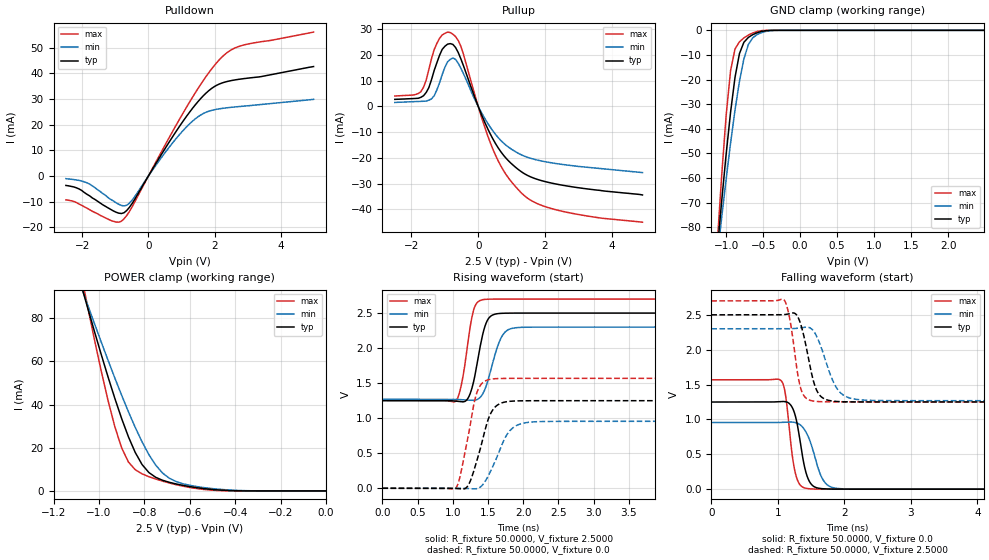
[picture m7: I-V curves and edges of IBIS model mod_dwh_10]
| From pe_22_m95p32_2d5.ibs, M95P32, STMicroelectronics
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|   Model mod_dwh_10
[Model]   mod_dwh_10
Model_type I/O
Polarity   Non-Inverting
Enable   Active-High
Vinl   =   0.750V
Vinh   =   1.750V
Vmeas  =   1.250V
Cref   =   30.0pF
C_comp   1.219pF   1.164pF   1.337pF
[Model Spec]
Vinl   0.750V  0.690V  0.810V  | <- for Vcc = 2.5V, 2.3V, 2.7V
Vinh   1.750V  1.610V  1.890V  | <- for Vcc = 2.5V, 2.3V, 2.7V
Vmeas  1.250V  1.150V  1.350V  | <- for Vcc = 2.5V, 2.3V, 2.7V
[Temperature Range]  25.0000   0.1050k   -40.0000
[Voltage Range]   2.5000V   2.3000V   2.7000V
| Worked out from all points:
|   slope of the pulldown table from 0 to 0.375 V, typ, clamps not added: 46.8 ohm
|   slope of the pullup table from 0 to 0.375 V, typ, clamps not added: 33.9 ohm
|   GND clamp passes 1 mA (typ) near -0.58 V on its own axis
|   POWER clamp passes 1 mA (typ) near -0.53 V on its own axis
|   rising waveform, R_fixture 50.0000, V_fixture 2.5000: 20-80 % time 148ps typ, 183ps min, 131ps max; typ from 1.25 V to 2.5 V
|   rising waveform, R_fixture 50.0000, V_fixture 0.0: 20-80 % time 210ps typ, 257ps min, 178ps max; typ from 0 V to 1.25 V
|   falling waveform, R_fixture 50.0000, V_fixture 0.0: 20-80 % time 144ps typ, 197ps min, 116ps max; typ from 1.25 V to 0 V
|   falling waveform, R_fixture 50.0000, V_fixture 2.5000: 20-80 % time 173ps typ, 240ps min, 135ps max; typ from 2.5 V to 1.25 V
[Pulldown]
|Voltage   I(typ)   I(min)   I(max)
-2.5V     -3.72mA    -1.07mA    -9.34mA
-1.86V    -7.2mA     -2.7mA     -12.6mA
-1.14V    -13.1mA    -9.2mA     -17.4mA
-820mV    -14.69mA   -11.52mA   -17.69mA
-660mV    -13.52mA   -11.47mA   -15.5mA
-500mV    -10.87mA   -9.532mA   -12.19mA
540mV     11.44mA    9.728mA    12.92mA
1.26V     25.15mA    20.5mA     29.15mA
1.74V     32.3mA     24.84mA    38.73mA
2.22V     36.25mA    26.34mA    46.35mA
2.86V     37.94mA    27.21mA    51.03mA
5V        42.7mA     29.9mA     56.16mA
[Pullup]
|Voltage   I(typ)   I(min)   I(max)
-2.5V     2.762mA    1.562mA    4.052mA
-1.72V    3.553mA    1.982mA    5.743mA
-1.48V    7.344mA    2.457mA    14.39mA
-1.24V    16.99mA    6.442mA    24.51mA
-1.08V    22.2mA     12.4mA     27.82mA
-840mV    24.44mA    18.28mA    28.74mA
-520mV    18.48mA    14.85mA    23.37mA
120mV     -3.865mA   -2.929mA   -5.077mA
520mV     -14.48mA   -10.9mA    -19.03mA
1.32V     -25.62mA   -18.96mA   -33.95mA
2.44V     -30.41mA   -22.38mA   -40.5mA
4.92V     -34.4mA    -25.7mA    -44.98mA
[GND_clamp]
|Voltage   I(typ)   I(min)   I(max)
-2.5V     -618.8mA   -507.1mA   -839.7mA
-1.12V    -89.51mA   -92.19mA   -86.51mA
-1.06V    -69.34mA   -76.02mA   -58.94mA
-1V       -50.38mA   -60.48mA   -34.64mA
-940mV    -33.28mA   -45.81mA   -16.38mA
-880mV    -19.11mA   -32.38mA   -7.564mA
-820mV    -9.453mA   -20.71mA   -4.67mA
-760mV    -4.854mA   -11.6mA    -3.093mA
-700mV    -2.891mA   -5.814mA   -1.933mA
-580mV    -964.2uA   -1.685mA   -447.5uA
-340mV    -4.19uA    -39.9uA    -134.6nA
2.48V     343.3pA    931.5nA    131.5pA
[POWER_clamp]
|Voltage   I(typ)   I(min)   I(max)
-2.49V    667.2mA    541mA      921mA
-1.08V    96.07mA    95.11mA    101.2mA
-1.05V    84.91mA    86.28mA    85.45mA
-990mV    63.23mA    68.98mA    55.57mA
-930mV    42.88mA    52.31mA    29.76mA
-900mV    33.53mA    44.31mA    19.96mA
-840mV    17.8mA     29.4mA     9.816mA
-810mV    12.22mA    22.72mA    7.905mA
-750mV    6.305mA    11.96mA    5.516mA
-660mV    3.226mA    4.34mA     2.89mA
-420mV    154.8uA    392.4uA    29.01uA
0V        492.2pA    14.11nA    240.5pA
[Ramp]
| variable   typ   min   max
dV/dt_r   0.7498/0.2355n   0.5900/0.3071n   0.9410/0.1910n
dV/dt_f   0.7496/0.2142n   0.6311/0.3208n   0.8690/0.1617n
R_load = 50.0000
[Rising Waveform]
R_fixture= 50.0000
V_fixture= 2.5000
V_fixture_min= 2.3000
V_fixture_max= 2.7000
|time   V(typ)   V(min)   V(max)
0s        1.251V     1.269V     1.252V
1.04ns    1.244V     1.268V     1.24V
1.136ns   1.233V     1.263V     1.547V
1.248ns   1.353V     1.256V     2.308V
1.312ns   1.597V     1.257V     2.59V
1.424ns   2.189V     1.345V     2.691V
1.52ns    2.438V     1.611V     2.699V
1.68ns    2.496V     2.132V     2.7V
1.872ns   2.5V       2.288V     2.7V
8ns       2.5V       2.3V       2.7V
[Rising Waveform]
R_fixture= 50.0000
V_fixture= 0.0
V_fixture_min= 0.0
V_fixture_max= 0.0
|time   V(typ)   V(min)   V(max)
0s        5.246nV    623.3nV    889pV
1.04ns    -2.183mV   587.5uV    -1.489mV
1.104ns   -7.264mV   -5.605nV   170.9mV
1.2ns     16.06mV    -2.904mV   644.9mV
1.344ns   399.9mV    -4.835mV   1.369V
1.424ns   692.4mV    48.27mV    1.506V
1.536ns   1.062V     240.9mV    1.556V
1.792ns   1.239V     797.6mV    1.568V
2.08ns    1.249V     941.7mV    1.568V
8ns       1.25V      955.1mV    1.568V
[Falling Waveform]
R_fixture= 50.0000
V_fixture= 0.0
V_fixture_min= 0.0
V_fixture_max= 0.0
|time   V(typ)   V(min)   V(max)
0s        1.25V      955.1mV    1.568V
1.056ns   1.258V     957.9mV    1.549V
1.12ns    1.253V     961.1mV    1.325V
1.216ns   1.173V     962.2mV    490.1mV
1.264ns   1.048V     955.2mV    228.3mV
1.424ns   235.5mV    817.6mV    12.35mV
1.52ns    53.72mV    586.1mV    2.853mV
1.664ns   7.123mV    161.3mV    372.6uV
1.888ns   595.9uV    11.41mV    22.35uV
8ns       1.028uV    1.623uV    1.112uV
[Falling Waveform]
R_fixture= 50.0000
V_fixture= 2.5000
V_fixture_min= 2.3000
V_fixture_max= 2.7000
|time   V(typ)   V(min)   V(max)
0s        2.5V       2.3V       2.7V
1.088ns   2.503V     2.299V     2.72V
1.184ns   2.519V     2.301V     2.418V
1.28ns    2.501V     2.306V     1.77V
1.344ns   2.365V     2.313V     1.447V
1.52ns    1.607V     2.286V     1.265V
1.648ns   1.329V     2.044V     1.254V
1.872ns   1.259V     1.469V     1.252V
2.16ns    1.251V     1.291V     1.252V
8ns       1.251V     1.269V     1.252V
